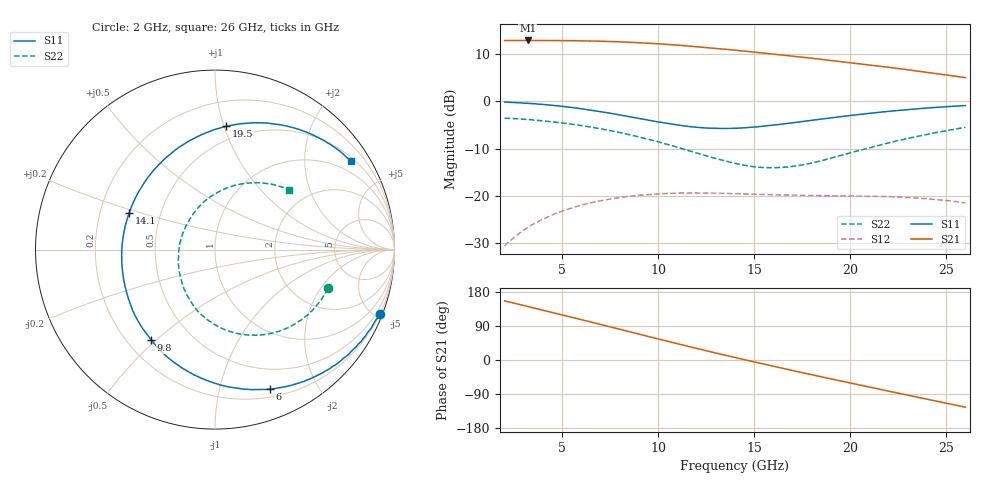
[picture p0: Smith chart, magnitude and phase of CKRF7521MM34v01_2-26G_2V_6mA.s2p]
! CHUO DENSHI KOGYO Co.,Ltd.
! 1. March 2016
! CKRF7521MM34
! N-channel HJ-FET
! Vds = 2 V Id = 6 mA
# Hz S  MA  R 50
!  f  S11  S21  S12  S22
!  Hz  MAG  ANG  MAG  ANG  MAG  ANG  MAG  ANG
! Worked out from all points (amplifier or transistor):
!   241 points, 2 GHz to 26 GHz, reference 50 ohm
!   highest |S21| = 12.9 dB at 3.2 GHz (marker M1)
!   |S21| within 3 dB of that: start of sweep to 16.23 GHz
!   unconditionally stable (mu >= 1): 13.68 GHz to 20.13 GHz
!   at 6 GHz: K = 0.44, MSG = 17.4 dB, |S12| = -22.0 dB
!   at 14 GHz: K = 1.02, MAG = 14.4 dB, |S12| = -19.5 dB
!   at 26 GHz: K = 0.61, MSG = 13.3 dB, |S12| = -21.5 dB
!   S11 on the Smith chart (normalised r, x): 2 GHz: 0.24, -5.32; 6 GHz: 0.28, -1.44; 9.8 GHz: 0.30, -0.48; 14.1 GHz: 0.33, +0.18; 19.5 GHz: 0.39, +1.01; 26 GHz: 0.60, +3.25
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2e9  0.9838 -21.3  4.419 155.9  0.02921 73.8  0.6641 -18.9
3.2e9  0.9552 -34.5  4.427 141.4  0.04614 63.7  0.6421 -30.6
4.8e9  0.8956 -53.3  4.419 121.7  0.06638 50.6  0.5984 -46.1
6e9  0.8353 -68.4  4.391 106.5  0.07948 40.8  0.5546 -58.1
7e9  0.7785 -81.8  4.345 93.8  0.08833 32.9  0.5127 -68.3
7.9e9  0.7247 -94.8  4.285 82.3  0.09508 25.7  0.4723 -77.8
8.8e9  0.6732 -108.6  4.209 70.9  0.1004 18.9  0.4299 -87.5
9.8e9  0.6165 -125.2  4.103 58.1  0.1041 11.6  0.3826 -98.6
1e10  0.6064 -128.5  4.079 55.6  0.1049 10.2  0.3733 -101.1
1.1e10  0.5624 -146.5  3.954 42.9  0.1066 3.4  0.3262 -113.2
1.2e10  0.5314 -164.9  3.804 30.6  0.1069 -2.6  0.2844 -126.0
1.3e10  0.5181 176.5  3.647 18.5  0.1064 -7.9  0.2484 -140.5
1.4e10  0.519 158.5  3.491 6.6  0.1053 -13.0  0.2207 -157.1
1.41e10  0.52 156.8  3.475 5.4  0.1051 -13.5  0.2186 -158.8
1.5e10  0.535 141.8  3.331 -5.1  0.1037 -17.2  0.2029 -175.2
1.6e10  0.5607 126.7  3.169 -16.5  0.1024 -21.1  0.1985 165.1
1.8e10  0.6297 100.9  2.868 -38.9  0.1004 -28.3  0.2225 128.2
1.95e10  0.6893 84.9  2.645 -55.3  0.09952 -33.6  0.2674 105.4
2.08e10  0.7402 72.7  2.462 -69.3  0.09896 -38.3  0.3143 88.8
2.2e10  0.7849 62.4  2.298 -82.2  0.09751 -43.4  0.3636 75.7
2.41e10  0.8534 46.3  2.022 -104.5  0.09233 -52.9  0.4524 55.4
2.6e10  0.9036 33.2  1.787 -124.6  0.08379 -62.2  0.5308 39.1
